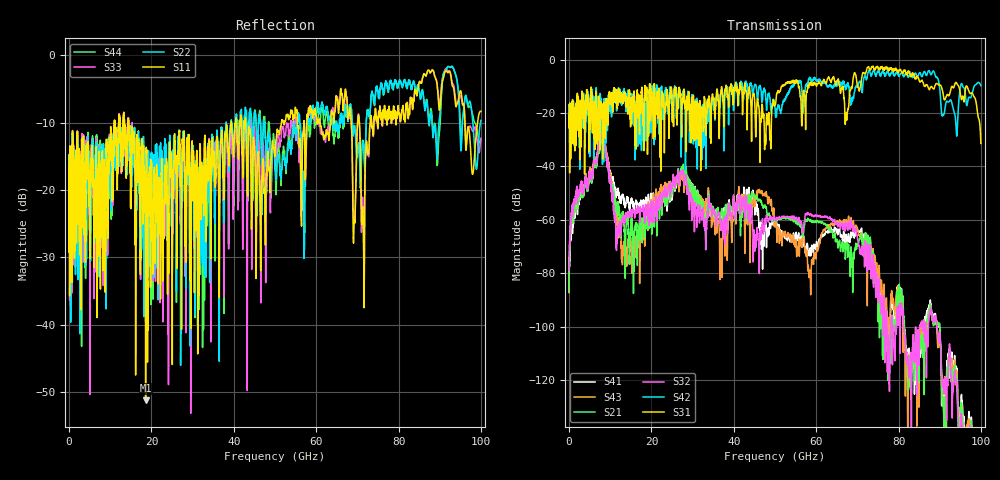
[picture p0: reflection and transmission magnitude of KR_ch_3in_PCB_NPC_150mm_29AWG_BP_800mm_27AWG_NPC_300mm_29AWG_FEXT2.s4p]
# GHz S RI R 45
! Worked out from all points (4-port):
!   4000 points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, 25 MHz to 100 GHz, reference 45 ohm
!   strongest paths, dB at 25 MHz, 25.02 GHz, 50.02 GHz, 75.03 GHz, 100 GHz:
!     S31: -21.2, -17.2, -16.7, -3.0, -31.4
!     S42: -21.3, -17.5, -18.0, -4.3, -9.8
!     S32: -78.9, -47.3, -59.8, -88.4, -145.9
!     S21: -86.7, -49.4, -60.3, -95.6, -148.3
!     S43: -87.1, -46.8, -59.5, -82.1, -139.6
!     S41: -87.2, -51.8, -60.3, -85.0, -139.7
!   lowest |S11| = -51.2 dB at 18.6 GHz (marker M1), VSWR 1.01, Z = 44.8 - j0.167 ohm
!   |S11| at or under -10 dB: start of sweep to 11.02 GHz; 14.46 GHz to 39.36 GHz (24.91 GHz wide, 92.6 % of centre); 42.94 GHz to 51.57 GHz (8.636 GHz wide, 18.3 % of centre)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
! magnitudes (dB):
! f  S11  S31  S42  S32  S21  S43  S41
! 25 MHz  -16.6  -21.2  -21.3  -78.9  -86.7  -87.1  -87.2
! 8.075 GHz  -15.2  -21.1  -21.6  -26.5  -28.6  -25.2  -27.3
! 13.15 GHz  -10.2  -13.5  -11.8  -60.0  -58.0  -71.5  -51.2
! 18.6 GHz  -51.2  -14.8  -21.1  -54.1  -55.6  -56.6  -51.8
! 27.62 GHz  -13.0  -14.6  -11.8  -42.9  -41.5  -45.3  -42.2
! 77.1 GHz  -9.6  -2.7  -5.1  -95.1  -104.2  -90.7  -95.1
! 100 GHz  -8.3  -31.4  -9.8  -145.9  -148.3  -139.6  -139.7
